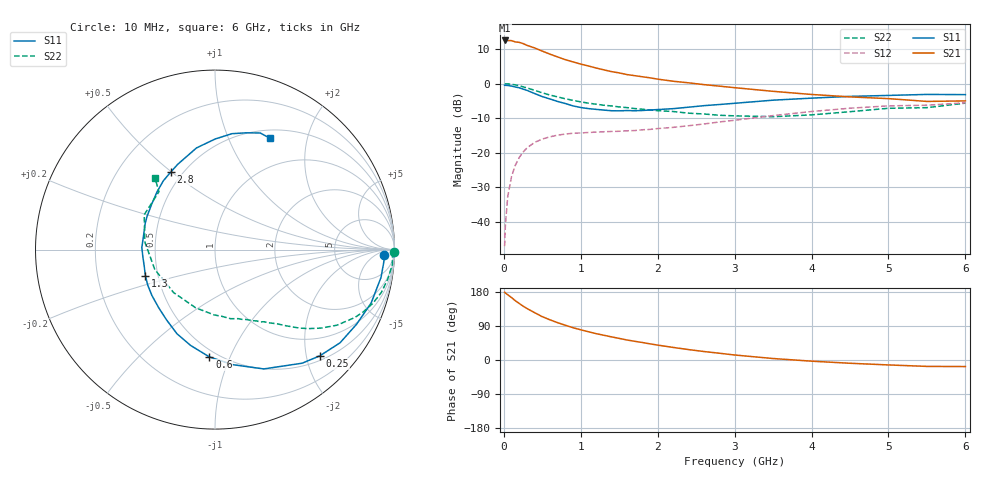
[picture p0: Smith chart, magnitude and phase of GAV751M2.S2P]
! Infineon Technologies  Discrete & RF Semiconductors
! BF775
! Si NPN RF Bipolar Junction Transistor in SOT23
! VCE = 0.75 V  IC = 1.2 mA
! Common Emitter S-Parameters:  May  1996
# GHz  S  MA  R  50
!  f  S11  S21  S12  S22
! GHz  MAG  ANG  MAG  ANG  MAG  ANG  MAG  ANG
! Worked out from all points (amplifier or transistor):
!   36 points, 10 MHz to 6 GHz, reference 50 ohm
!   highest |S21| = 12.4 dB at 10 MHz (marker M1)
!   |S21| within 3 dB of that: start of sweep to 491.3 MHz
!   unconditionally stable (mu >= 1): 1.251 GHz to end of sweep
!   at 250 MHz: K = 0.24, MSG = 15.7 dB, |S12| = -19.8 dB
!   at 1.4 GHz: K = 1.09, MAG = 6.8 dB, |S12| = -13.8 dB
!   at 6 GHz: K = 1.09, MAG = -1.6 dB, |S12| = -5.6 dB
!   S11 on the Smith chart (normalised r, x): 10 MHz: 27, -14; 250 MHz: 0.59, -2.26; 600 MHz: 0.45, -0.84; 1.3 GHz: 0.43, -0.15; 2.8 GHz: 0.43, +0.50; 6 GHz: 0.60, +1.43
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0.01  0.9437 -1.8  4.187 178.8  0.0045 88.7  0.9975 -0.9
0.02  0.9434 -4.0  4.121 176.8  0.0089 87.2  0.9894 -2.0
0.05  0.938 -9.5  4.174 172.3  0.0231 83.3  0.9915 -4.9
0.1  0.9195 -18.9  4.166 164.7  0.0455 78.1  0.9763 -9.8
0.15  0.8916 -27.8  3.986 156.3  0.0665 72.5  0.9573 -14.4
0.2  0.869 -36.7  3.933 149.2  0.0855 67.3  0.9297 -18.7
0.25  0.8314 -45.4  3.773 142.2  0.1022 62.3  0.8967 -22.7
0.3  0.7978 -52.5  3.562 136.0  0.1177 58.3  0.865 -26.0
0.4  0.7181 -67.8  3.265 124.9  0.1415 50.9  0.7994 -31.8
0.5  0.648 -81.4  2.937 114.3  0.1582 44.7  0.7352 -36.5
0.6  0.5986 -93.0  2.655 106.0  0.1704 40.1  0.6819 -40.2
0.8  0.5146 -114.3  2.208 91.6  0.1867 33.5  0.6028 -45.4
0.9  0.4758 -124.5  2.051 85.2  0.1918 31.3  0.5721 -47.6
1.1  0.4347 -143.9  1.793 74.5  0.1967 28.5  0.5216 -51.9
1.3  0.414 -159.6  1.577 65.3  0.2016 27.0  0.4866 -55.7
1.6  0.4078 178.3  1.348 52.8  0.2081 26.8  0.4497 -61.8
2.2  0.434 144.4  1.08 33.2  0.2331 29.5  0.3949 -77.2
2.8  0.4981 119.5  0.918 17.9  0.2789 30.9  0.3487 -99.2
3.5  0.5758 100.3  0.772 3.9  0.345 27.4  0.3324 -134.0
4.5  0.6527 81.7  0.642 -8.6  0.4409 16.3  0.3926 174.0
5.5  0.6969 68.8  0.552 -16.9  0.4868 2.1  0.4489 134.1
6  0.692 63.8  0.562 -17.3  0.5278 -1.9  0.5217 129.9
